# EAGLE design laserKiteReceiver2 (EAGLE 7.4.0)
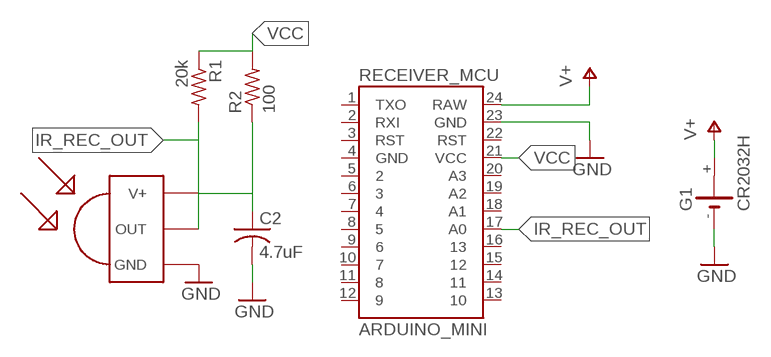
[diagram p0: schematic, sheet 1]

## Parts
C2  4.7uF  C-US025-025X050  [C025-025X050]
G1  CR2032H  [CR2032H]
R1  20k  R-US_0309/V  [0309V]
R2  100  R-US_0309/V  [0309V]
RECEIVER_MCU  ARDUINO_MINI  [ARDUINO_MINI]
U$1  TSOP1738  [TSOP17XX]

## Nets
GND: C2.2 G1.- RECEIVER_MCU.23(GND) U$1.GND
IR_REC_OUT: R1.2 RECEIVER_MCU.17(A0) U$1.OUT
N$1: C2.1 R2.1 U$1.V+
V+: G1.+ RECEIVER_MCU.24(RAW)
VCC: R1.1 R2.2 RECEIVER_MCU.21(VCC)
Unconnected: G1.+@1(+) RECEIVER_MCU.1(TXO) RECEIVER_MCU.2(RXI) RECEIVER_MCU.3(RST) RECEIVER_MCU.4(GND) RECEIVER_MCU.5 RECEIVER_MCU.6 RECEIVER_MCU.7 RECEIVER_MCU.8 RECEIVER_MCU.9 RECEIVER_MCU.10 RECEIVER_MCU.11 RECEIVER_MCU.12 RECEIVER_MCU.13 RECEIVER_MCU.14 RECEIVER_MCU.15 RECEIVER_MCU.16 RECEIVER_MCU.18(A1) RECEIVER_MCU.19(A2) RECEIVER_MCU.20(A3) RECEIVER_MCU.22(RST)

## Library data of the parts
C2 = adafruit:C-US: CAPACITOR, American symbol
G1 = battery:CR2032H: LI BATTERY Varta
R1 R2 = adafruit:R-US_: RESISTOR, American symbol
RECEIVER_MCU = SparkFun-Boards:ARDUINO_MINI: Arduino Pro Mini footprint
U$1 = tsop:TSOP1738: IR Receiver and Demodulator

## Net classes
0 default: width 1.016 mm, drill 0.508 mm, clearance 0.508 mm

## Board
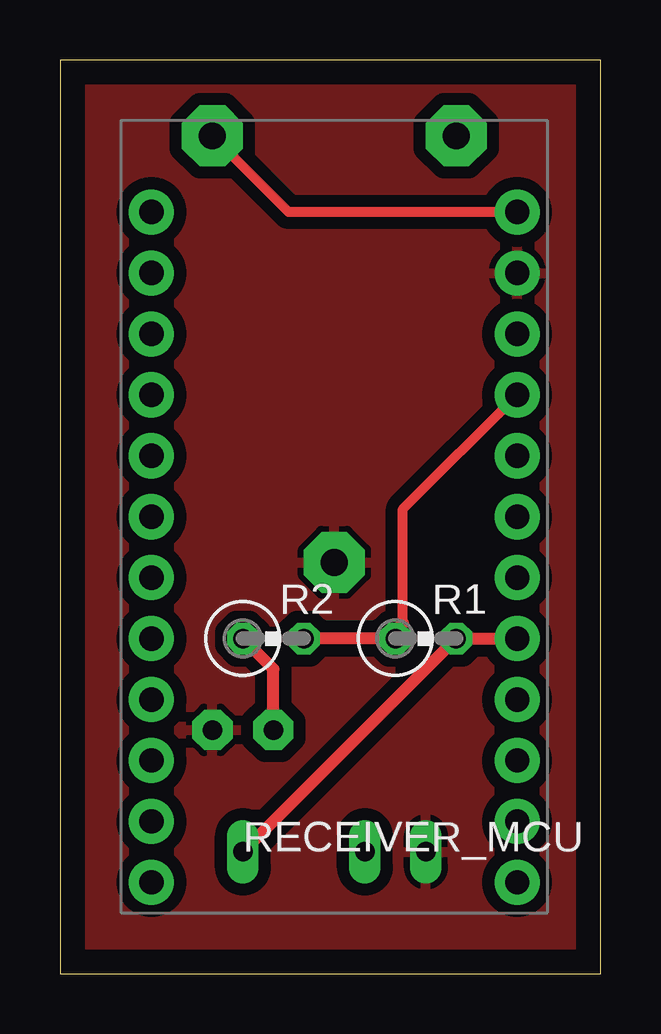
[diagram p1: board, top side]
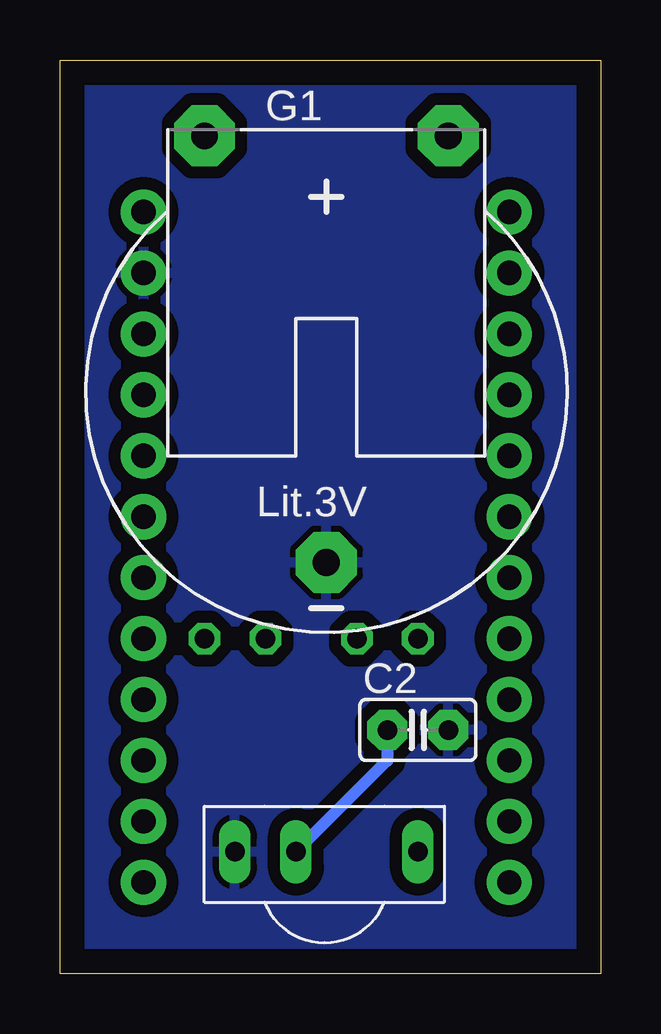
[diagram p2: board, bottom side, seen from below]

Size 22.53 x 38.09 mm. Coordinates in mm from the lower left corner, seen from the top.
Outline: 0,0 22.53,0 22.53,38.09 0,38.09 0,0
Copper layers (1*16): Top 0.035mm / dielectric 1.5mm / Bottom 0.035mm
Design rules "default": minimum track width 10mil, minimum drill 24mil, track to track 8mil, track to pad 8mil, pad to pad 8mil, via to via 8mil, smd to smd 8mil, copper to edge 40mil, drill to drill 8mil, minimum pad ring 10mil, minimum via ring 8mil, stop-mask expansion 4mil, vias tented up to drill 0mil, thermal gap 10mil

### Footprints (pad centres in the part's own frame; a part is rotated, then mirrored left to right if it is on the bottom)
C025-025X050 = drill 0.813 pad 1.676 octagon: 1 -1.27,0; 2 1.27,0
CR2032H = drill 1.118 pad 2.54 octagon: + 5.08,10.795; +@1 -5.08,10.795; - 0,-6.985
0309V = drill 0.813 octagon: 1 -1.27,0; 2 1.27,0
ARDUINO_MINI = drill 1.016 pad 1.88: 1 -7.62,12.7; 2 -7.62,10.16; 3 -7.62,7.62; 4 -7.62,5.08; 5 -7.62,2.54; 6 -7.62,0; 7 -7.62,-2.54; 8 -7.62,-5.08; 9 -7.62,-7.62; 10 -7.62,-10.16; 11 -7.62,-12.7; 12 -7.62,-15.24; 13 7.62,-15.24; 14 7.62,-12.7; 15 7.62,-10.16; 16 7.62,-7.62; 17 7.62,-5.08; 18 7.62,-2.54; 19 7.62,0; 20 7.62,2.54; 21 7.62,5.08; 22 7.62,7.62; 23 7.62,10.16; 24 7.62,12.7
TSOP17XX = drill 0.813 long: GND -3.81,0; OUT 3.81,0; V+ -1.27,0

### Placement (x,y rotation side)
C2  7.62,10.16 0 bottom
G1  11.43,24.13 0 bottom
R1  15.24,13.97 0 top
R2  8.89,13.97 0 top
RECEIVER_MCU  11.43,19.05 0 top
U$1  11.43,5.08 0 bottom

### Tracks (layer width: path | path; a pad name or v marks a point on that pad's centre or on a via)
GND
  pour Top: -1.27,39.37 60.96,39.37 60.96,-1.27 -1.27,-1.27
  pour Bottom: -1.27,39.37 60.96,39.37 60.96,-1.27 -1.27,-1.27
IR_REC_OUT
  Top 0.508: U$1.OUT R1.2 RECEIVER_MCU.17
N$1
  Top 0.508: R2.1 8.89,12.7 C2.1
  Bottom 0.508: U$1.V+ 8.89,8.89 C2.1
V+
  Top 0.406: RECEIVER_MCU.24 9.53,31.75 G1.+
VCC
  Top 0.406: 14.29,14.61 14.29,19.37 RECEIVER_MCU.21
  Top 0.508: R2.2 R1.1 13.97,14.29 14.29,14.61

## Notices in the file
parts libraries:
SparkFun-Boards: Licensing: Creative Commons ShareAlike 4.0 International - https://creativecommons.org/licenses/by-sa/4.0
